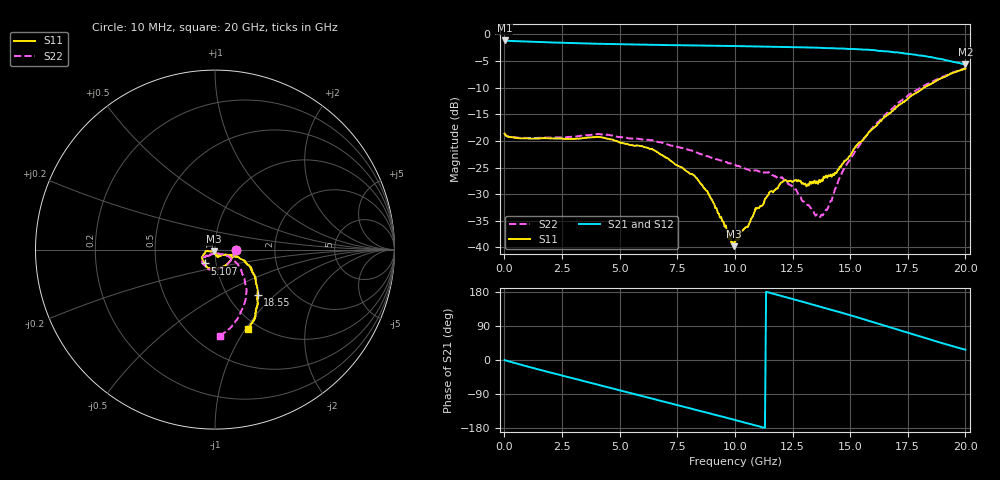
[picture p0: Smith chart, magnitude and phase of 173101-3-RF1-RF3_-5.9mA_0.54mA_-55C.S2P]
!  2-Port S-parameters saved by WinCal
! VAR MeasName=S-Parameters (CALIBRATED_DATA) read from VNA (N5242A)
! VAR MeasDate=2017-7-20 10:27:31
! VAR NAME=173101-3-RF1-RF3_-5.9mA_0.54mA_-55C
! VAR FILENAME=173101-3-RF1-RF3_-5.9mA_0.54mA_-55C.S2P
! VAR DATE=2017-7-20 10:27:31
! VAR PHYS_PORTS=1,2
# Hz S DB R 50
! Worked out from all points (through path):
!   401 points, 10 MHz to 20 GHz, reference 50 ohm
!   highest |S21| = -1.13 dB at 10 MHz (marker M1); lowest = -5.6 dB at 20 GHz (marker M2)
!   group delay of S21, straight-line fit = 45.7 ps
!   lowest |S11| = -39.8 dB at 9.955 GHz (marker M3), VSWR 1.02, Z = 49.5 - j0.891 ohm
!   |S11| at or under -10 dB: start of sweep to 18.2 GHz
!   |S22| runs from -34.3 to -6.3 dB; largest |S21 - S12| = 0.0086
!   S11 on the Smith chart (normalised r, x): 10 MHz: 1.26, -0.01; 5.107 GHz: 0.88, -0.14; 18.55 GHz: 1.36, -0.79; 20 GHz: 0.90, -1.03
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1e7  -18.63 -2.3  -1.13 -0.1  -1.13 -0.2  -18.60 -2.4
1.559225e9  -19.53 -52.2  -1.43 -26.1  -1.44 -26.1  -19.40 -50.5
3.358325e9  -19.51 -96.1  -1.67 -54.4  -1.68 -54.4  -19.00 -91.0
4.157925e9  -19.29 -112.6  -1.76 -66.7  -1.77 -66.8  -18.73 -106.6
5.10745e9  -20.38 -126.6  -1.84 -81.4  -1.86 -81.5  -19.31 -117.3
6.70665e9  -22.34 -152.1  -1.96 -106.3  -1.96 -106.2  -20.24 -136.8
8.30585e9  -26.87 -170.1  -2.08 -131.2  -2.09 -131.1  -22.08 -146.9
8.90555e9  -30.36 -161.3  -2.11 -140.7  -2.12 -140.6  -23.04 -143.7
9.855075e9  -39.26 -125.6  -2.17 -155.8  -2.18 -155.9  -24.29 -146.0
9.955025e9  -39.78 -118.7  -2.18 -157.4  -2.20 -157.5  -24.42 -145.5
1.0005e10  -38.80 -118.8  -2.19 -158.3  -2.21 -158.3  -24.53 -145.6
1.090455e10  -32.60 -79.1  -2.25 -172.7  -2.27 -172.7  -25.54 -136.7
1.205398e10  -27.77 -71.9  -2.35 168.5  -2.36 168.5  -26.83 -132.9
1.335332e10  -27.68 -52.4  -2.48 146.6  -2.45 146.6  -32.88 -102.6
1.36032e10  -28.06 -45.1  -2.49 142.4  -2.50 142.2  -33.96 -96.6
1.390305e10  -26.93 -45.3  -2.56 137.4  -2.56 137.2  -33.56 -76.6
1.430285e10  -26.41 -35.8  -2.61 130.3  -2.63 130.3  -29.68 -45.1
1.485258e10  -23.50 -24.5  -2.70 120.6  -2.71 120.6  -24.36 -29.3
1.590205e10  -17.99 -18.5  -2.92 101.6  -2.93 101.2  -17.86 -30.7
1.670165e10  -14.77 -21.6  -3.22 86.9  -3.29 86.4  -14.40 -39.2
1.855072e10  -9.17 -47.0  -4.28 52.5  -4.37 52.6  -8.90 -64.5
2e10  -6.39 -67.2  -5.64 27.1  -5.69 27.8  -6.33 -86.7
